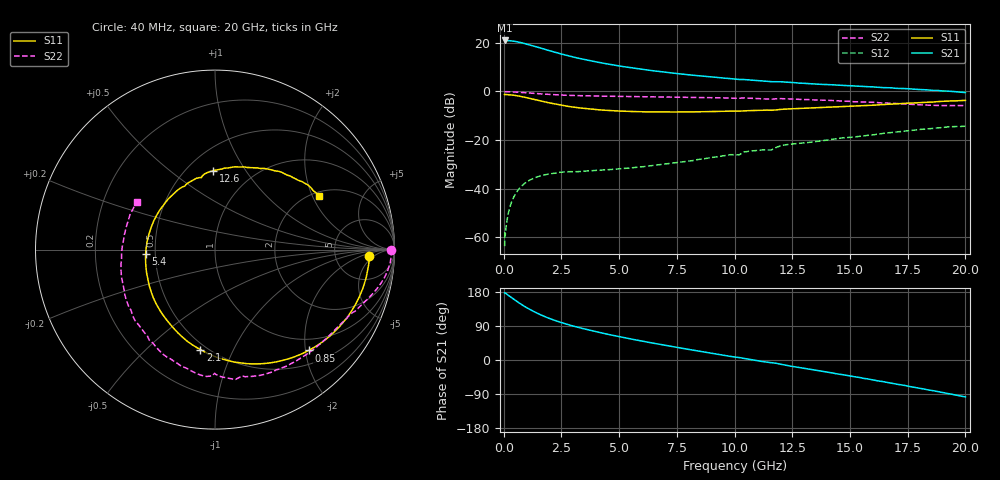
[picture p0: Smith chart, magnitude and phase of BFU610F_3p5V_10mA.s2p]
! Filename:  P:\Prog\Test\Noise\ATS_data\Testdata_Net\SplitFiles\BFU610_2W_A5_HighFreq_3.5V_10mA_D.s2p
! Date/Time: Wed 10/Aug/2011 16:56:41
! BFU610_2W_A5_HighFreq_Bias4_3.5V_1mA_10mA_R.s2p
! MDIF S-parameter v. bias file
! BFU610_2W_A5_HighFreq_3.5V_1mA_10mA
! Date/time Mon Aug 08 14:10:09 2011
! VAR V_out= 3.5010
! VAR I_out= 9.9900
! VAR V_in= 0.9107
! VAR I_in= 0.0918
! Device data file deembeded for feedlines and parallel
! Original file: \SplitFiles\BFU610_2W_A5_HighFreq_3.5V_10mA_R.s2p
! Feed-files: PR003V01_101208_Feed1.s2p, PR003V01_101208_Feed2.s2p
! Parallel-file: PR003V01_101208_Par.s2p
# MHz S MA R 50
!  Freq-MHz  S11-mag  S11-arg  S21-mag  S21-arg  S12-mag  S12-arg  S22-mag  S22-arg
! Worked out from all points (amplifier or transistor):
!   167 points, 40 MHz to 20 GHz, reference 50 ohm
!   highest |S21| = 20.9 dB at 40 MHz (marker M1)
!   |S21| within 3 dB of that: start of sweep to 1.555 GHz
!   unconditionally stable (mu >= 1): 2.824 GHz to end of sweep
!   at 550 MHz: K = 0.20, MSG = 31.0 dB, |S12| = -41.6 dB
!   at 4.2 GHz: K = 1.50, MAG = 17.9 dB, |S12| = -32.4 dB
!   at 20 GHz: K = 1.14, MAG = 4.7 dB, |S12| = -14.3 dB
!   S11 on the Smith chart (normalised r, x): 40 MHz: 13, -3; 850 MHz: 0.76, -2.06; 2.1 GHz: 0.46, -0.75; 5.4 GHz: 0.44, -0.03; 12.6 GHz: 0.66, +0.73; 20 GHz: 2.16, +2.25
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40  0.8608 -2.2  11.09 177.6  0.0006605 76.7  0.9798 -0.1
50  0.8537 -2.8  11.05 177.6  0.001337 87.5  0.9808 -0.3
70  0.861 -4.0  11.03 176.6  0.001104 82.2  0.9824 -0.7
260  0.8507 -15.1  10.96 168.1  0.00407 81.9  0.9798 -3.7
400  0.8363 -23.1  10.77 161.9  0.006185 78.0  0.9739 -5.8
600  0.8089 -34.2  10.37 153.3  0.009076 72.2  0.9614 -8.5
850  0.7664 -47.2  9.735 143.5  0.0122 65.1  0.9426 -11.6
1100  0.7211 -59.1  9.06 134.5  0.01475 59.2  0.9232 -14.2
1350  0.6766 -70.2  8.383 126.5  0.01678 54.2  0.9043 -16.6
1750  0.6114 -86.1  7.375 115.3  0.01913 47.9  0.8778 -19.9
2100  0.5627 -98.3  6.599 106.9  0.02048 43.9  0.8595 -22.7
2700  0.4984 -116.8  5.524 95.0  0.0223 39.3  0.8305 -26.6
3400  0.451 -134.8  4.61 83.5  0.02279 38.1  0.8126 -31.2
4300  0.4111 -155.0  3.793 70.6  0.02423 39.0  0.7967 -37.1
5400  0.3874 -176.1  3.114 56.8  0.02652 42.7  0.7828 -44.6
6800  0.3767 160.8  2.532 40.9  0.03124 47.4  0.7671 -54.4
8800  0.3838 132.8  2.014 19.7  0.04207 51.0  0.7469 -69.0
10200  0.3917 115.5  1.753 6.5  0.04958 52.6  0.7217 -78.4
12600  0.4404 91.2  1.508 -17.8  0.08354 42.8  0.6912 -100.4
13400  0.4572 83.4  1.42 -25.7  0.09142 38.2  0.6678 -108.2
16800  0.5464 54.2  1.181 -61.2  0.1426 15.1  0.5683 -150.4
20000  0.6528 27.3  0.9451 -97.5  0.1921 -17.9  0.5099 148.9
